(* Logix 5000 AddOnInstructionDefinition export AMCI_NXFE2_Jog_CCW; software revision 20.03 *)

ADD_ON_INSTRUCTION AMCI_NXFE2_Jog_CCW   (* revision 1.0, vendor AMCI, ExecuteEnableInFalse *)
VAR_INPUT
   Axis_Status_Bits : DINT; {required}
        .1   // Set when moving CCW
   _0_normal_1_S_curve_acceleration : BOOL;
   _0_Triangular_1_Trapezoidal_S_Curve : BOOL;
   Programmed_Speed : DINT; {required}
   Acceleration : INT; {required}
   Deceleration : INT; {required}
END_VAR
VAR_IN_OUT
   NXFE2_output_data : _000A:NXFE2_0986AEB4:O:0; {required}
END_VAR
VAR_OUTPUT
   EN : BOOL; {access Read Only, visible}
   Jog_CCW_Occurring : BOOL; {access Read Only, visible}
   ER : BOOL; {access Read Only, visible}
END_VAR
VAR
   command_data_block : INT[10];
        [0]   // Command Bits MSW
        [1]   // Command Bits LSW
        [3]   // Lower Target Position
        [4]   // Upper Programmed Speed
        [5]   // Lower Programmed Speed
END_VAR

ROUTINE EnableInFalse   (* ladder *)
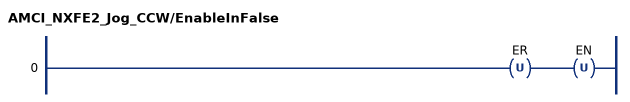
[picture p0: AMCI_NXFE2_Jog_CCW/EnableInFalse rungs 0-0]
   0: OTU(ER)OTU(EN);
END_ROUTINE

ROUTINE Logic   (* ladder *)
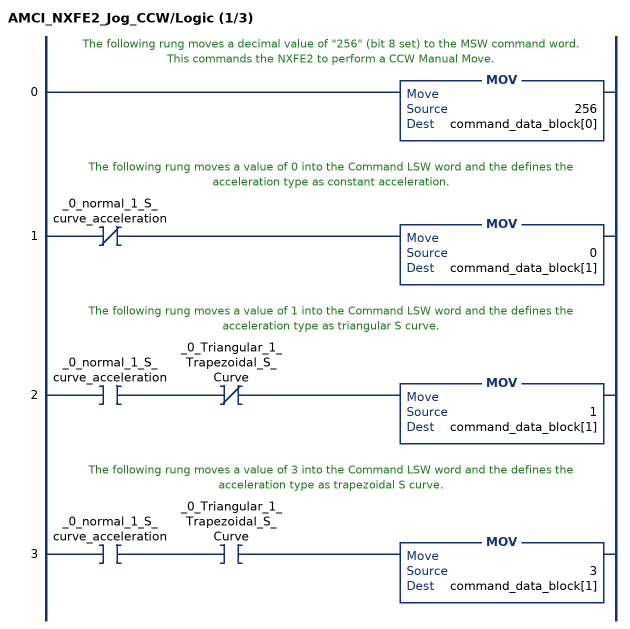
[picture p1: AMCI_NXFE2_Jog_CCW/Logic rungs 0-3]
   // The following rung moves a decimal value of "256" (bit 8 set) to the MSW command word.  This commands the NXFE2 to perform a CCW Manual Move.
   0: MOV(256,command_data_block[0]);
   // The following rung moves a value of 0 into the Command LSW word and the defines the acceleration type as constant acceleration.
   1: XIO(_0_normal_1_S_curve_acceleration)MOV(0,command_data_block[1]);
   // The following rung moves a value of 1 into the Command LSW word and the defines the acceleration type as triangular S curve.
   2: XIC(_0_normal_1_S_curve_acceleration)XIO(_0_Triangular_1_Trapezoidal_S_Curve)MOV(1,command_data_block[1]);
   // The following rung moves a value of 3 into the Command LSW word and the defines the acceleration type as trapezoidal S curve.
   3: XIC(_0_normal_1_S_curve_acceleration)XIC(_0_Triangular_1_Trapezoidal_S_Curve)MOV(3,command_data_block[1]);
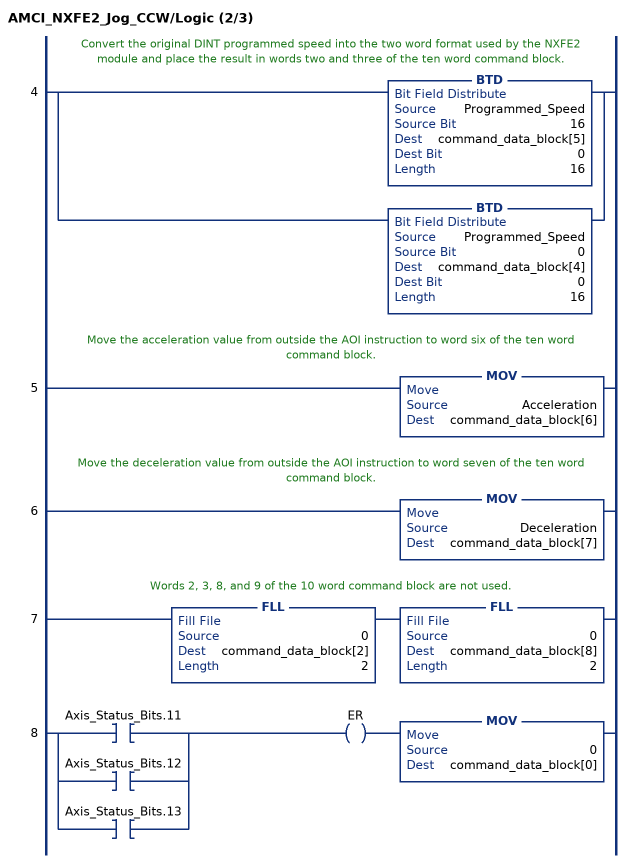
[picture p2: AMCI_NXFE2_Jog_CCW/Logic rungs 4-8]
   // Convert the original DINT programmed speed into the two word format used by the NXFE2 module and place the result in words two and three of the ten word command block.
   4: [BTD(Programmed_Speed,16,command_data_block[5],0,16) ,BTD(Programmed_Speed,0,command_data_block[4],0,16) ];
   // Move the acceleration value from outside the AOI instruction to word six of the ten word command block.
   5: MOV(Acceleration,command_data_block[6]);
   // Move the deceleration value from outside the AOI instruction to word seven of the ten word command block.
   6: MOV(Deceleration,command_data_block[7]);
   // Words 2, 3, 8, and 9 of the 10 word command block are not used.
   7: FLL(0,command_data_block[2],2)FLL(0,command_data_block[8],2);
   8: [XIC(Axis_Status_Bits.11) ,XIC(Axis_Status_Bits.12) ,XIC(Axis_Status_Bits.13) ]OTE(ER)MOV(0,command_data_block[0]);
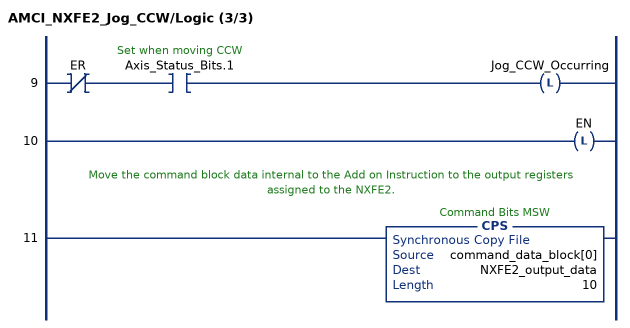
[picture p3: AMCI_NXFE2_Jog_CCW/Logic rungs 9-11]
   9: XIO(ER)XIC(Axis_Status_Bits.1)OTL(Jog_CCW_Occurring);
   10: OTL(EN);
   // Move the command block data internal to the Add on Instruction to the output registers assigned to the NXFE2.
   11: CPS(command_data_block[0],NXFE2_output_data,10);
END_ROUTINE
END_ADD_ON_INSTRUCTION
